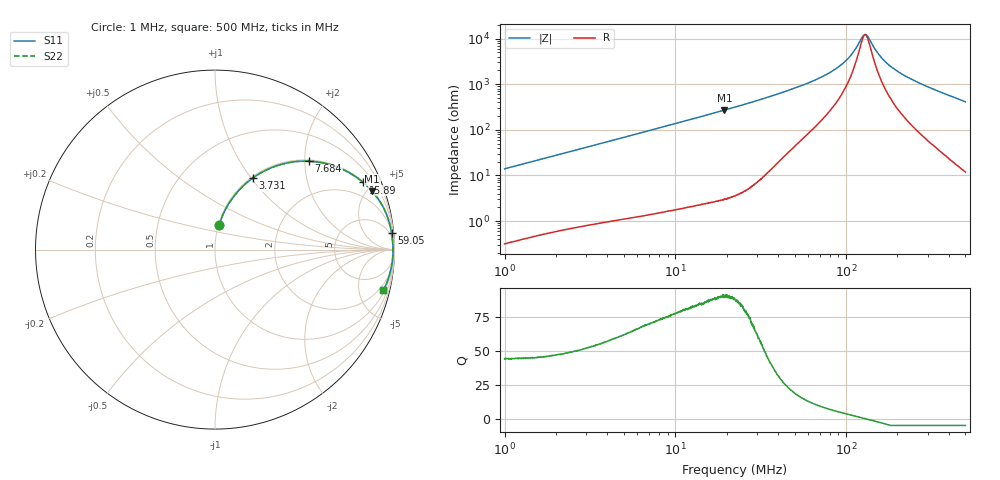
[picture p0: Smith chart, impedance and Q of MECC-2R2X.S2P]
!s-Parameter Generated by FASTRON Sdn. Bhd.
!FASTRON P/N : MECC-2R2X
!Keysight Technologies,E4991B,MY54100416,A.01.15
!Date: Wed Apr 01 14:55:30 2026
!Version  : Rev00 Wed Apr 01 14:55:30 2026
!Data & Calibration Information:
!PortZ  Port1:50+j0  Port2:50+j0
!When reading, reference impedance value at option line is always used.
!Remarks : This data is being provided solely for informational purposes.
!Freq	S11	S21	S12	S22
# Hz S dB R 50
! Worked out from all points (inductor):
!   1601 points, 1 MHz to 500 MHz, reference 50 ohm
!   read as one part in series: L = 2.21 uH near 1.032 MHz
!   highest Q = 90.5 at 19.37 MHz (marker M1), where L = 2.22 uH
!   self-resonance near 129.5 MHz
!   S11 on the Smith chart (normalised r, x): 1 MHz: 1.01, +0.28; 3.731 MHz: 1.02, +1.02; 7.684 MHz: 1.03, +2.10; 15.89 MHz: 1.05, +4.38; 59.05 MHz: 3, +21; 500 MHz: 1.24, -8.22
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1000000  -17.22 80.8  -0.11 -7.9  -0.11 -7.9  -17.22 80.8
2820919  -8.90 67.8  -0.67 -21.0  -0.67 -21.0  -8.90 67.8
3731163  -6.90 62.1  -1.07 -26.9  -1.07 -26.9  -6.90 62.1
7684215  -2.87 43.2  -3.29 -46.0  -3.29 -46.0  -2.87 43.2
7957584  -2.72 42.3  -3.45 -47.0  -3.45 -47.0  -2.72 42.3
1.588699e7  -0.86 24.4  -7.68 -64.9  -7.68 -64.9  -0.86 24.4
1.93674e7  -0.59 20.3  -9.20 -69.1  -9.20 -69.1  -0.59 20.3
2.236068e7  -0.45 17.6  -10.39 -71.8  -10.39 -71.8  -0.45 17.6
3.792254e7  -0.17 9.8  -15.36 -78.6  -15.36 -78.6  -0.17 9.8
5.904717e7  -0.10 5.4  -20.42 -80.2  -20.42 -80.2  -0.10 5.4
6.307767e7  -0.10 4.9  -21.31 -80.1  -21.31 -80.1  -0.10 4.9
8.02529e7  -0.08 3.1  -25.17 -78.6  -25.17 -78.6  -0.08 3.1
9.632587e7  -0.08 1.9  -29.33 -74.4  -29.33 -74.4  -0.08 1.9
1.082302e8  -0.07 1.1  -33.31 -66.8  -33.31 -66.8  -0.07 1.1
1.239906e8  -0.07 0.3  -40.53 -30.2  -40.53 -30.2  -0.07 0.3
1.289013e8  -0.07 0.0  -41.84 -3.6  -41.84 -3.6  -0.07 0.0
1.34528e8  -0.07 -0.2  -40.79 27.4  -40.79 27.4  -0.07 -0.2
1.577516e8  -0.07 -1.3  -32.53 69.0  -32.53 69.0  -0.07 -1.3
1.77937e8  -0.07 -2.1  -28.54 75.7  -28.54 75.7  -0.07 -2.1
2.086543e8  -0.08 -3.2  -24.86 79.0  -24.86 79.0  -0.08 -3.2
2.563485e8  -0.10 -4.9  -21.29 80.0  -21.29 80.0  -0.10 -4.9
5e8  -0.31 -13.6  -12.58 74.8  -12.58 74.8  -0.31 -13.6
